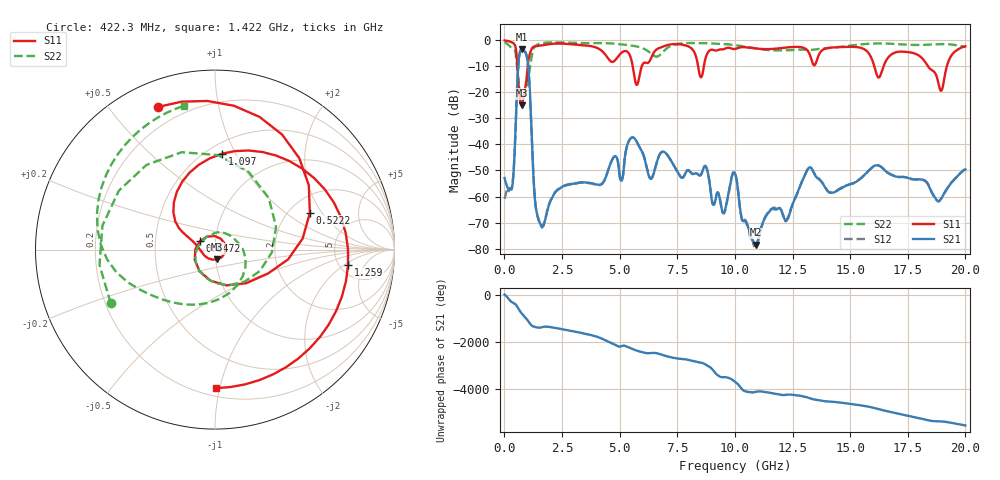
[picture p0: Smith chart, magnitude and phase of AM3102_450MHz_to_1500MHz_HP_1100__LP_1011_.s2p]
!Agilent Technologies,E8364B,MY43040894,A.07.50.67
!Agilent E8364B: A.07.50.67
!Date: Thursday, January 11, 2018 06:35:03
!Correction: S11(Full 2 Port(1,2))
!S21(Full 2 Port(1,2))
!S12(Full 2 Port(1,2))
!S22(Full 2 Port(1,2))
!S2P File: Measurements: S11, S21, S12, S22:
# Hz S  dB  R 50
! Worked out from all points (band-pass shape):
!   1601 points, 10 MHz to 20 GHz, reference 50 ohm
!   highest |S21| = -3.53 dB at 772.1 MHz (marker M1); lowest = -78.5 dB at 10.9 GHz (marker M2)
!   |S21| within 3 dB of the highest: 636.8 MHz to 980.8 MHz (344.1 MHz wide, 42.5 % of centre)
!   lowest |S11| = -25.0 dB at 747.1 MHz (marker M3), VSWR 1.12, Z = 50.9 - j5.61 ohm
!   |S11| at or under -10 dB: 560.9 MHz to 1.011 GHz (450.2 MHz wide, 57.3 % of centre); 5.567 GHz to 5.962 GHz (394.9 MHz wide, 6.85 % of centre); 18.38 GHz to 19.2 GHz (818.7 MHz wide, 4.36 % of centre)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
!   |S22| runs from -21.6 to -0.7 dB; largest |S21 - S12| = 0.0014
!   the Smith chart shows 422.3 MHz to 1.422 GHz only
!   S11 on the Smith chart (normalised r, x): 422.3 MHz: 0.11, +0.67; 522.2 MHz: 2.57, +1.55; 647.2 MHz: 0.84, +0.08; 1.097 GHz: 0.59, +0.88; 1.259 GHz: 5.93, -2.35; 1.422 GHz: 0.26, -0.98
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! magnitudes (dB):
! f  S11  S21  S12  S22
! 10 MHz  -0.1  -52.9  -60.9  -0.7
! 422.3 MHz  -1.4  -47.2  -46.9  -3.7
! 522.2 MHz  -4.9  -24.6  -24.5  -7.6
! 647.2 MHz  -20.4  -5.8  -5.8  -18.8
! 747.1 MHz  -25.0  -3.6  -3.6  -21.1
! 772.1 MHz  -24.2  -3.5  -3.5  -21.0
! 1.097 GHz  -5.4  -18.3  -18.3  -11.2
! 1.259 GHz  -2.5  -51.9  -51.9  -3.3
! 1.422 GHz  -2.2  -66.8  -67.1  -1.7
! 3.346 GHz  -1.9  -54.7  -54.6  -1.1
! 5.082 GHz  -4.8  -53.9  -54.0  -1.6
! 5.745 GHz  -17.1  -39.0  -39.0  -2.4
! 6.332 GHz  -7.5  -53.2  -53.0  -4.9
! 6.682 GHz  -3.1  -45.0  -44.9  -6.1
! 8.731 GHz  -6.8  -48.3  -48.3  -1.1
! 9.505 GHz  -3.5  -66.3  -66.4  -1.4
! 10.01 GHz  -3.4  -51.1  -51.2  -1.9
! 10.9 GHz  -3.2  -78.5  -78.6  -3.1
! 13.34 GHz  -8.0  -49.4  -49.4  -3.7
! 16.68 GHz  -6.4  -51.1  -51.0  -1.3
! 18.94 GHz  -19.4  -61.0  -60.9  -1.5
! 20 GHz  -2.3  -49.6  -49.4  -2.5
